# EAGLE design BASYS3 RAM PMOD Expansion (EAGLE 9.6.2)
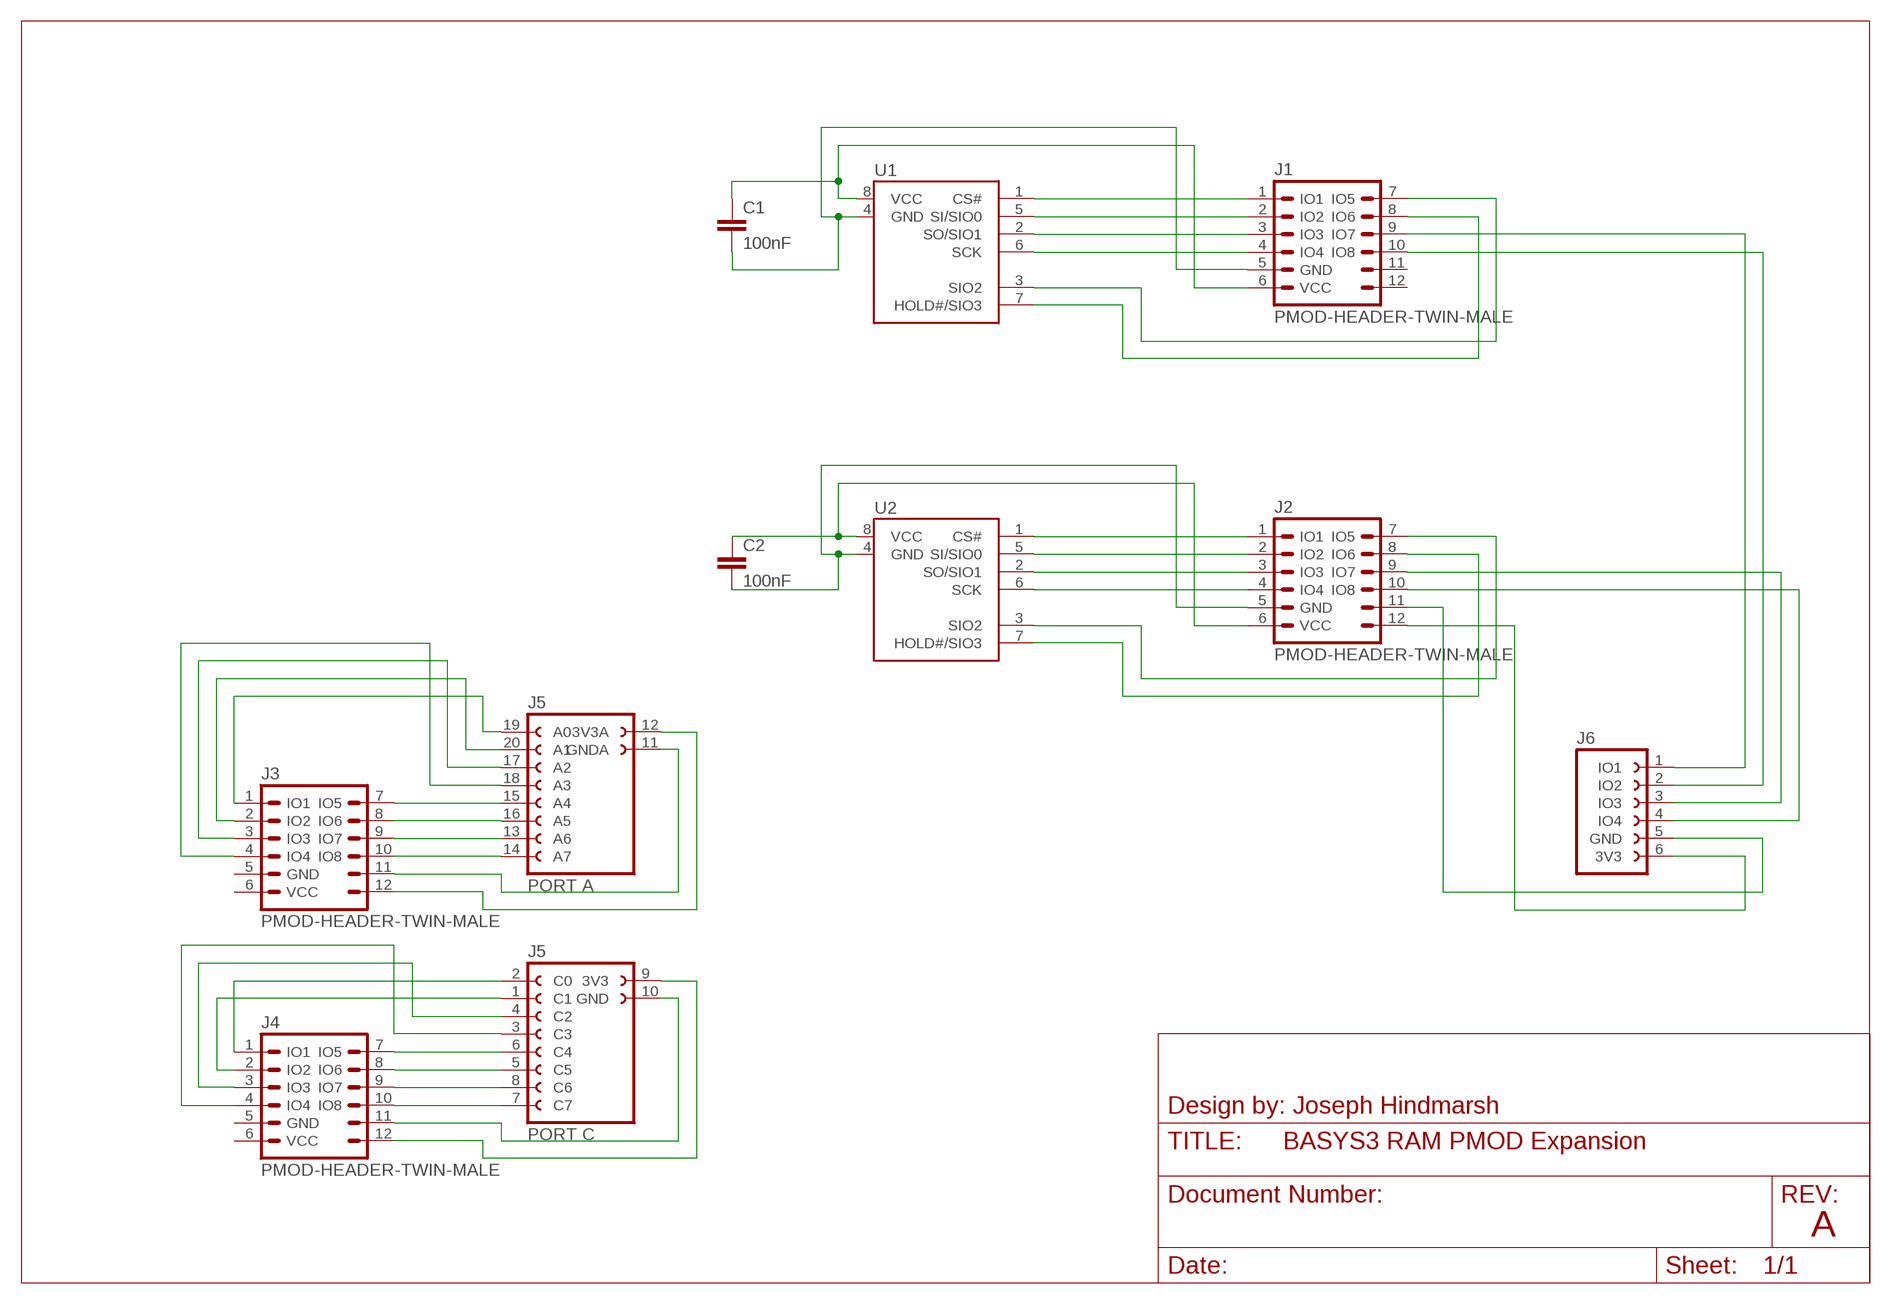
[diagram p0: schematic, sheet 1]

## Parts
C1  100nF  C-EU050-025X075  [C050-025X075]
C2  100nF  C-EU050-025X075  [C050-025X075]
J1  PMOD-HEADER-TWIN-MALE  [MA06-2W-PMOD]
J2  PMOD-HEADER-TWIN-MALE  [MA06-2W-PMOD]
J3  PMOD-HEADER-TWIN-MALE  [MA06-2W-PMOD]
J4  PMOD-HEADER-TWIN-MALE  [MA06-2W-PMOD]
J5  IL-MATTO-TWIN-HEADER  [FE05-2-IL-MATTO]
J6  PMOD-HEADER-FEMALE  [FE06W]
U1  23LC1024DIP  [DIL08]
U2  23LC1024DIP  [DIL08]

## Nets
N$1: J1.1(IO1) U1.1(CS#)
N$2: J1.2(IO2) U1.5(SI/SIO0)
N$3: J1.3(IO3) U1.2(SO/SIO1)
N$4: J1.4(IO4) U1.6(SCK)
N$5: J1.7(IO5) U1.3(SIO2)
N$6: J1.8(IO6) U1.7(HOLD#/SIO3)
N$7: C1.2 J1.5(GND) U1.4(GND)
N$8: C1.1 J1.6(VCC) U1.8(VCC)
N$9: J2.1(IO1) U2.1(CS#)
N$10: J2.2(IO2) U2.5(SI/SIO0)
N$11: J2.3(IO3) U2.2(SO/SIO1)
N$12: J2.4(IO4) U2.6(SCK)
N$13: J2.7(IO5) U2.3(SIO2)
N$14: J2.8(IO6) U2.7(HOLD#/SIO3)
N$15: C2.2 J2.5(GND) U2.4(GND)
N$16: C2.1 J2.6(VCC) U2.8(VCC)
N$17: J2.12(VCC2) J6.6(3V3)
N$18: J2.11(GND2) J6.5(GND)
N$19: J1.9(IO7) J6.1(IO1)
N$20: J1.10(IO8) J6.2(IO2)
N$21: J2.9(IO7) J6.3(IO3)
N$22: J2.10(IO8) J6.4(IO4)
N$23: J3.1(IO1) J5.19(A0)
N$24: J3.10(IO8) J5.14(A7)
N$25: J3.9(IO7) J5.13(A6)
N$26: J3.8(IO6) J5.16(A5)
N$27: J3.7(IO5) J5.15(A4)
N$28: J3.4(IO4) J5.18(A3)
N$29: J3.2(IO2) J5.20(A1)
N$30: J3.3(IO3) J5.17(A2)
N$31: J4.10(IO8) J5.7(C7)
N$32: J4.9(IO7) J5.8(C6)
N$33: J4.8(IO6) J5.5(C5)
N$34: J4.7(IO5) J5.6(C4)
N$35: J4.4(IO4) J5.3(C3)
N$36: J4.3(IO3) J5.4(C2)
N$37: J4.2(IO2) J5.1(C1)
N$38: J4.1(IO1) J5.2(C0)
N$39: J3.11(GND2) J5.11(GNDA)
N$40: J3.12(VCC2) J5.12(3V3A)
N$41: J4.11(GND2) J5.10(GND)
N$42: J4.12(VCC2) J5.9(3V3)

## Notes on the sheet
- Design by: Joseph Hindmarsh
- A

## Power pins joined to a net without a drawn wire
GND: J3.5(GND) J4.5(GND)
GND2: J1.11(GND2)
VCC: J3.6(VCC) J4.6(VCC)
VCC2: J1.12(VCC2)

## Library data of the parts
C1 C2 = rcl:C-EU: CAPACITOR, European symbol; SPICEPREFIX: C
J1-J4 = joe_lib:PMOD-HEADER-TWIN-MALE
J5 = joe_lib:IL-MATTO-TWIN-HEADER
J6 = joe_lib:PMOD-HEADER-FEMALE: FEMALE HEADER; OC_FARNELL: unknown; OC_NEWARK: unknown
U1 U2 = joe_lib:23LC1024: 23LC1024 QSPI 1Mbit SRAM 1Mbit Serial SRAM

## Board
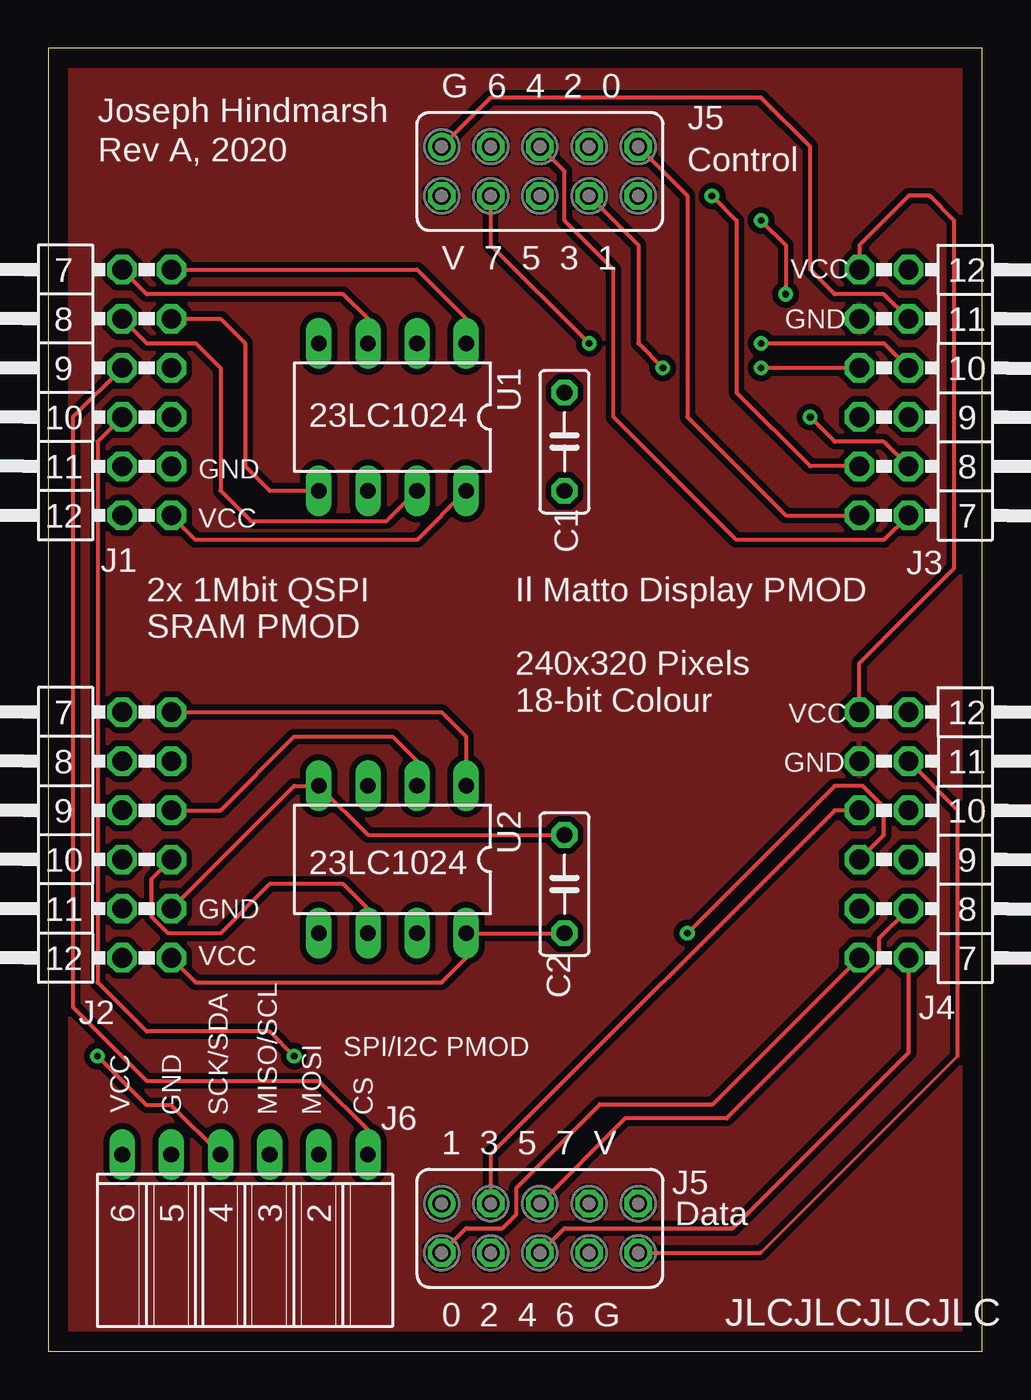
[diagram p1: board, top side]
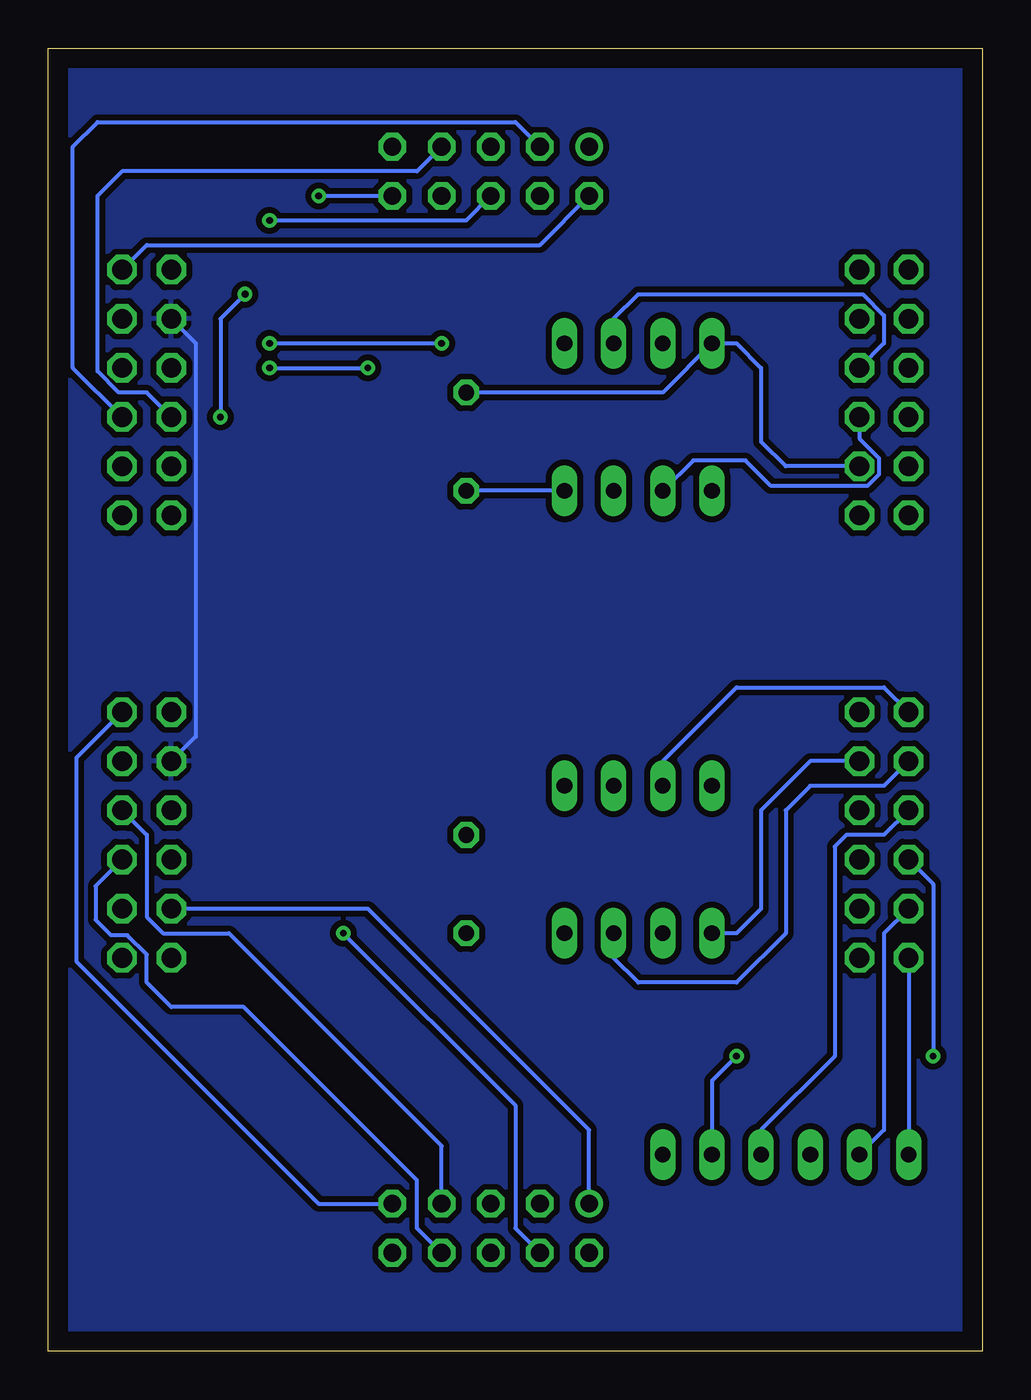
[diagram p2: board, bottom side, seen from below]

Size 48.26 x 67.31 mm. Coordinates in mm from the lower left corner, seen from the top.
Outline: 0,0 48.26,0 48.26,67.31 0,67.31 0,0
Copper layers (1*16): Top 0.035mm / dielectric 1.5mm / Bottom 0.035mm
Design rules "default": minimum track width 6mil, minimum drill 0.35mm, track to track 6mil, track to pad 6mil, pad to pad 6mil, via to via 6mil, smd to smd 6mil, copper to edge 40mil, drill to drill 6mil, minimum pad ring 10mil, minimum via ring 8mil, stop-mask expansion 4mil, vias tented up to drill 0mil, thermal gap 10mil

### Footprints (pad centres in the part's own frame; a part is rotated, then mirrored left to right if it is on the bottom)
C050-025X075 = drill 0.813 octagon: 1 -2.54,0; 2 2.54,0
MA06-2W-PMOD = drill 1.016 octagon: 1 5.08,-1.27; 2 2.54,-1.27; 3 0,-1.27; 4 -2.54,-1.27; 5 -5.08,-1.27; 6 -7.62,-1.27; 7 5.08,1.27; 8 2.54,1.27; 9 0,1.27; 10 -2.54,1.27; 11 -5.08,1.27; 12 -7.62,1.27
FE05-2-IL-MATTO = drill 0.914: 1 -5.08,1.27; 11 -5.08,55.88 | drill 0.914 octagon: 2 -5.08,-1.27; 3 -2.54,1.27; 4 -2.54,-1.27; 5 0,1.27; 6 0,-1.27; 7 2.54,1.27; 8 2.54,-1.27; 9 5.08,1.27; 10 5.08,-1.27; 12 -5.08,53.34; 13 -2.54,55.88; 14 -2.54,53.34; 15 0,55.88; 16 0,53.34; 17 2.54,55.88; 18 2.54,53.34; 19 5.08,55.88; 20 5.08,53.34
FE06W = drill 0.813 long: 1 -6.35,0; 2 -3.81,0; 3 -1.27,0; 4 1.27,0; 5 3.81,0; 6 6.35,0
DIL08 = drill 0.813 long: 1 -3.81,-3.81; 2 -1.27,-3.81; 3 1.27,-3.81; 4 3.81,-3.81; 5 3.81,3.81; 6 1.27,3.81; 7 -1.27,3.81; 8 -3.81,3.81

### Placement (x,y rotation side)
C1  26.67,46.99 90 top
C2  26.67,24.13 90 top
J1  5.08,50.8 90 top
J2  5.08,27.94 90 top
J3  43.18,48.26 270 top
J4  43.18,25.4 270 top
J5  25.4,6.35 0 top
J6  10.16,10.16 180 top
U1  17.78,48.26 180 top
U2  17.78,25.4 180 top

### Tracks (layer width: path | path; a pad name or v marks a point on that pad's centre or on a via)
GND
  Bottom 0.203: J4.5 40.64,31.75 40.64,52.07 J3.5
  pour Top (isolate 0.305): 0,67.31 48.26,67.31 48.26,0 0,0
  pour Bottom (isolate 0.305): 0,67.31 48.26,67.31 48.26,0 0,0
N$1
  Top 0.203: U1.1 21.59,53.34 19.05,55.88 J1.1
N$2
  Top 0.203: J1.2 8.89,53.34 10.16,52.07 10.16,45.72 11.43,44.45 U1.5
N$3
  Bottom 0.203: U1.2 19.05,53.34 17.78,54.61 6.18,54.61 5.08,53.51 5.08,52.07 J1.3
N$4
  Bottom 0.203: U1.6 14.94,46.03 12.24,46.03 10.92,44.7 5.93,44.7 5.33,45.3 5.33,46.14 6.35,47.16 J1.4
N$5
  Top 0.203: U1.3 16.51,53.34 15.24,54.61 5.08,54.61 J1.7
N$6
  Top 0.203: J1.8 5.08,52.07 7.62,52.07 8.89,50.8 8.89,44.45 10.46,42.88 17.48,42.88 U1.7
N$7
  Bottom 0.203: C1.2 16.51,49.53 U1.4 12.7,52.07 11.43,50.8 11.43,46.99 10.16,45.72 J1.5
N$8
  Top 0.203: J1.6 7.62,41.91 19.05,41.91 U1.8
  Bottom 0.203: U1.8 C1.1
N$9
  Top 0.203: J2.1 20.32,33.02 21.59,31.75 U2.1
N$10
  Bottom 0.203: J2.2 8.89,30.48 11.43,27.94 11.43,22.86 12.7,21.59 U2.5
N$11
  Top 0.203: J2.3 8.89,27.94 12.7,31.75 17.78,31.75 19.05,30.48 U2.2
N$12
  Top 0.203: U2.6 16.51,22.86 15.24,24.13 11.43,24.13 8.89,21.59 6.18,21.59 5.33,22.44 5.33,24.38 J2.4
N$13
  Bottom 0.203: U2.3 16.51,30.48 12.7,34.29 5.08,34.29 J2.7
N$14
  Bottom 0.203: J2.8 5.08,29.21 8.89,29.21 10.16,27.94 10.16,21.59 12.7,19.05 17.78,19.05 19.05,20.32 U2.7
N$15
  Top 0.203: C2.2 16.51,26.67 U2.4 12.7,29.21 J2.5
N$16
  Top 0.203: C2.1 U2.8 21.59,20.32 20.32,19.05 7.62,19.05 J2.6
N$17
  Bottom 0.203: J2.12 J6.6
N$18
  Bottom 0.203: J2.11 5.08,21.59 5.08,11.43 J6.5
N$19
  Top 0.203: J1.9 1.27,48.26 1.27,17.78 5.08,13.97 13.97,13.97 16.51,11.43 J6.1
N$20  (via drill 0.35)
  Top 0.203: J1.10 2.54,46.99 2.54,19.05 5.08,16.51 11.43,16.51 v12.7,15.24
  Bottom 0.203: v12.7,15.24 13.97,13.97 J6.2
N$21
  Bottom 0.203: J2.9 5.08,26.67 7.03,26.67 7.62,26.07 7.62,15.24 11.43,11.43 J6.3
N$22  (via drill 0.35)
  Top 0.203: J6.4 6.35,12.7 5.08,12.7 v2.54,15.24
  Bottom 0.203: J2.10 2.54,24.13 v2.54,15.24
N$23
  Top 0.203: J5.19 33.02,59.69 33.02,48.26 38.1,43.18 J3.1
N$24  (via drill 0.35)
  Top 0.203: v27.94,52.07 22.86,57.15 J5.14 | v36.83,52.07 43.18,52.07 J3.10
  Bottom 0.203: v36.83,52.07 v27.94,52.07
N$25
  Bottom 0.203: J5.13 24.13,63.5 45.72,63.5 46.99,62.23 46.99,50.8 J3.9
N$26  (via drill 0.35)
  Top 0.203: v36.83,58.42 38.1,57.15 v38.1,54.61 | v39.37,48.26 40.64,46.99 43.18,46.99 J3.8
  Bottom 0.203: J5.16 26.67,58.42 v36.83,58.42 | v38.1,54.61 39.37,53.34 v39.37,48.26
N$27
  Top 0.203: J3.7 43.18,41.91 35.56,41.91 29.21,48.26 29.21,55.88 26.67,58.42 26.67,60.96 J5.15
N$28  (via drill 0.35)
  Top 0.203: J3.4 v36.83,50.8 | J5.18 30.48,57.15 30.48,52.07 v31.75,50.8
  Bottom 0.203: v36.83,50.8 v31.75,50.8
N$29  (via drill 0.35)
  Top 0.203: J3.2 39.37,45.72 35.56,49.53 35.56,58.42 v34.29,59.69
  Bottom 0.203: v34.29,59.69 J5.20
N$30
  Bottom 0.203: J5.17 29.21,60.96 44.45,60.96 45.72,59.69 45.72,50.63 44.62,49.53 43.18,49.53 J3.3
N$31
  Bottom 0.203: J5.7 27.94,10.6 38.93,21.59 42.33,21.59 43.18,22.44 43.18,26.67 J4.10
N$32
  Bottom 0.203: J4.9 45.82,24.03 45.82,22.29 45.02,21.49 44.18,21.49 43.18,20.49 43.18,19.05 41.91,17.78 38.16,17.78 29.21,8.83 29.21,6.35 J5.8
N$33
  Top 0.203: J4.8 42.93,21.34 42.93,19.9 35.04,12.01 29.79,12.01 J5.5
N$34
  Top 0.203: J4.7 44.45,15.43 35.37,6.35 26.67,6.35 J5.6
N$35
  Top 0.203: J4.4 40.64,27.94 22.86,10.16 J5.3
N$36  (via drill 0.35)
  Top 0.203: v33.02,21.59 40.64,29.21 42.08,29.21 43.18,28.11 43.18,26.67 J4.3
  Bottom 0.203: J5.4 24.13,6.35 24.13,12.7 v33.02,21.59
N$37
  Bottom 0.203: J5.1 20.32,11.43 31.75,22.86 J4.2
N$38
  Top 0.203: J4.1 34.34,12.75 28.5,12.75 24.18,8.43 24.18,7.07 23.46,6.35 21.59,6.35 J5.2
N$39
  Top 0.203: J5.11 22.86,64.77 36.83,64.77 39.37,62.23 39.37,55.88 40.64,54.61 43.18,54.61 J3.11
N$40
  Bottom 0.203: J3.12 43.18,57.15 22.86,57.15 J5.12
N$41
  Top 0.152: 36.82,5.08 46.99,15.25
  Top 0.203: J5.10 36.82,5.08 | J4.11 46.99,27.94 46.99,15.25
N$42
  Bottom 0.203: J4.12 46.81,30.66 46.81,20.14 34.29,7.62 J5.9
VCC
  Top 0.203: J4.6 41.91,35.56 46.81,40.46 46.81,58.42 45.54,59.69 44.45,59.69 41.91,57.15 J3.6

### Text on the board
tPlace: Joseph Hindmarsh | Rev A, 2020 | Control | VCC | GND | 23LC1024 | GND | VCC | 2x 1Mbit QSPI / SRAM PMOD | Il Matto Display PMOD / / 240x320 Pixels / 18-bit Colour | VCC | GND | 23LC1024 | GND | VCC | SPI/I2C PMOD | VCC | GND | SCK/SDA | MISO/SCL | MOSI | CS | Data | JLCJLCJLCJLC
